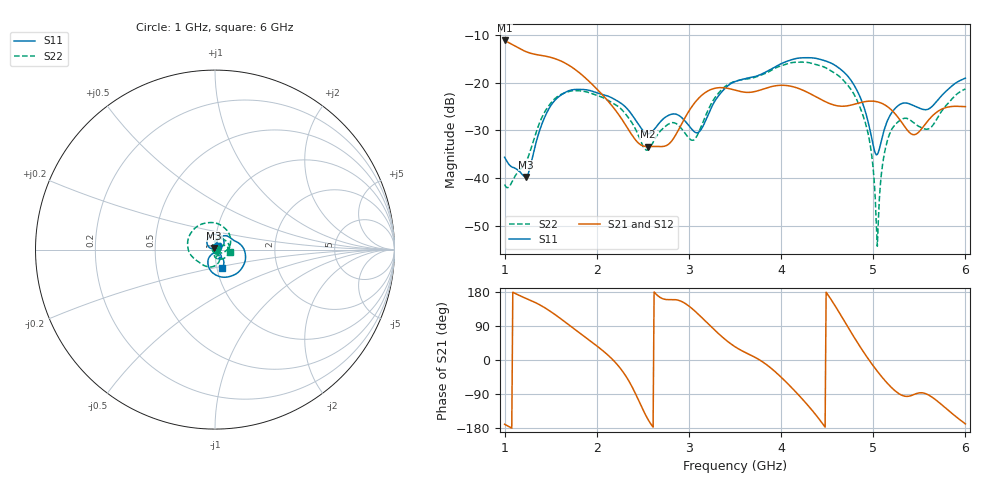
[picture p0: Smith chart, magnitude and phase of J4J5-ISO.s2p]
!Agilent Technologies,E8364B,MY43040528,A.07.50.67
!Agilent E8364B: A.07.50.67
!Date: Sunday, March 01, 2026 21:03:37
!Correction: S11(Full 2 Port(1,2))
!S21(Full 2 Port(1,2))
!S12(Full 2 Port(1,2))
!S22(Full 2 Port(1,2))
!S2P File: Measurements: S11, S21, S12, S22:
# Hz S  dB  R 50
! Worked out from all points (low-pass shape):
!   451 points, 1 GHz to 6 GHz, reference 50 ohm
!   highest |S21| = -11.21 dB at 1 GHz (marker M1); lowest = -33.4 dB at 2.556 GHz (marker M2)
!   |S21| within 3 dB of the highest: start of sweep to 1.358 GHz
!   lowest |S11| = -39.7 dB at 1.233 GHz (marker M3), VSWR 1.02, Z = 49.4 + j0.852 ohm
!   |S11| at or under -10 dB: start of sweep to end of sweep
!   |S22| runs from -54.2 to -15.7 dB; largest |S21 - S12| = 0.00092
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1e9  -35.63 59.5  -11.21 -169.6  -11.24 -169.6  -41.32 36.0
1.233333e9  -39.74 123.2  -13.56 162.4  -13.59 162.3  -36.66 99.1
1.5e9  -24.86 141.7  -14.74 127.8  -14.76 127.8  -24.35 74.1
1.844444e9  -21.46 81.8  -18.49 65.7  -18.51 65.8  -21.80 -5.0
2.255556e9  -24.24 34.6  -27.20 -21.9  -27.22 -21.9  -25.36 -74.7
2.555556e9  -30.72 41.4  -33.41 -156.6  -33.45 -156.6  -34.09 -72.9
2.666667e9  -28.75 56.2  -33.38 168.7  -33.41 168.7  -30.69 -56.8
2.855556e9  -26.61 42.1  -30.99 159.1  -31.02 159.1  -28.53 -82.5
3.055556e9  -30.24 43.8  -24.42 131.1  -24.45 131.1  -31.98 -72.1
3.288889e9  -23.64 73.3  -21.18 76.8  -21.21 76.9  -23.00 -71.3
3.5e9  -19.80 47.2  -21.59 35.0  -21.62 35.1  -19.77 -111.1
4.344444e9  -14.85 -44.5  -22.63 -135.0  -22.66 -134.9  -16.06 110.5
4.644444e9  -17.21 -90.6  -24.95 119.8  -24.99 119.8  -18.93 42.7
4.844444e9  -22.47 -121.6  -24.28 39.9  -24.32 39.9  -24.62 -9.3
4.966667e9  -30.11 -124.3  -23.89 -4.2  -23.92 -4.1  -32.98 -46.1
5.044444e9  -35.05 -76.8  -24.04 -29.7  -24.07 -29.7  -54.22 -159.7
5.1e9  -31.27 -46.9  -24.42 -46.5  -24.45 -46.5  -37.32 109.4
5.166667e9  -27.45 -42.3  -25.22 -64.9  -25.26 -64.9  -31.32 86.5
5.311111e9  -24.38 -57.4  -28.40 -93.1  -28.43 -93.0  -27.67 47.8
5.444444e9  -24.88 -67.5  -30.91 -90.8  -30.94 -90.8  -28.51 23.9
5.611111e9  -25.42 -55.9  -27.61 -93.8  -27.64 -93.8  -29.61 29.5
6e9  -19.08 -70.2  -25.05 -168.6  -25.08 -168.6  -21.32 -8.1
